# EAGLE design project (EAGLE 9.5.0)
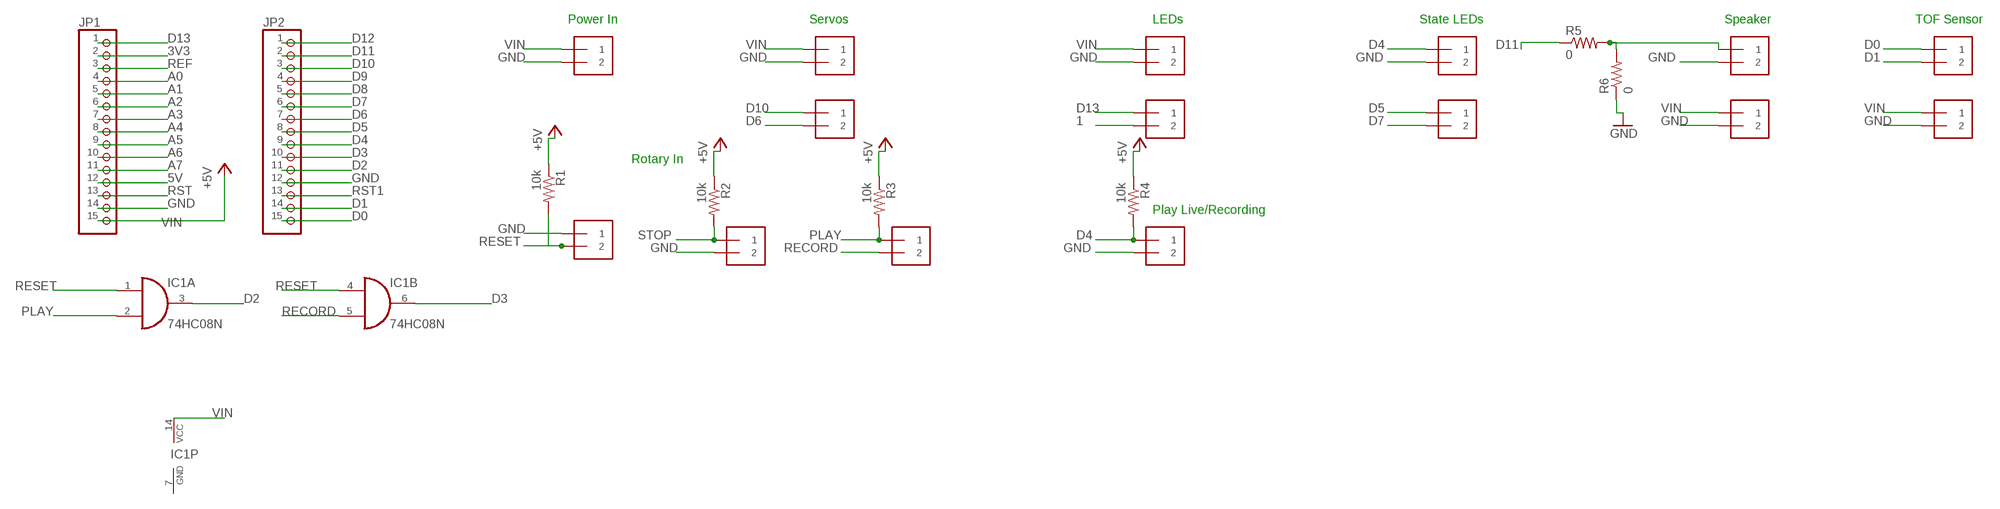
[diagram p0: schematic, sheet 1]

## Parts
IC1  74HC08N  [DIL14]
J1  1X2-3.5MM  [1X2-3.5MM]
J2  1X2-3.5MM  [1X2-3.5MM]
J3  1X2-3.5MM  [1X2-3.5MM]
J4  1X2-3.5MM  [1X2-3.5MM]
JP1  PINHD-1X15  [1X15]
JP2  PINHD-1X15  [1X15]
LED1  1X2-3.5MM  [1X2-3.5MM]
LED2_3  1X2-3.5MM  [1X2-3.5MM]
LED_PWR  1X2-3.5MM  [1X2-3.5MM]
LED_SIG  1X2-3.5MM  [1X2-3.5MM]
POWER  1X2-3.5MM  [1X2-3.5MM]
R1  10k  R-US_M0805  [M0805]
R2  10k  R-US_M0805  [M0805]
R3  10k  R-US_M0805  [M0805]
R4  10k  R-US_M0805  [M0805]
R5  0  R-US_M0805  [M0805]
R6  0  R-US_M0805  [M0805]
SERVO_PWR  1X2-3.5MM  [1X2-3.5MM]
SERVO_SIG  1X2-3.5MM  [1X2-3.5MM]
SPK_PWR  1X2-3.5MM  [1X2-3.5MM]
SPK_SIG  1X2-3.5MM  [1X2-3.5MM]
TOF_PWR  1X2-3.5MM  [1X2-3.5MM]
TOF_SIG  1X2-3.5MM  [1X2-3.5MM]

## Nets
1: LED_SIG.2
3V3: JP1.2
5V: JP1.12
A0: JP1.4
A1: JP1.5
A2: JP1.6
A3: JP1.7
A4: JP1.8
A5: JP1.9
A6: JP1.10
A7: JP1.11
D0: JP2.15 TOF_SIG.1
D1: JP2.14 TOF_SIG.2
D2: IC1.3(A:O) JP2.11
D3: IC1.6(B:O) JP2.10
D4: J1.1 JP2.9 LED1.1 R4.2
D5: JP2.8 LED2_3.1
D6: JP2.7 SERVO_SIG.2
D7: JP2.6 LED2_3.2
D8: JP2.5
D9: JP2.4
D10: JP2.3 SERVO_SIG.1
D11: JP2.2 R5.1
D12: JP2.1
D13: JP1.1 LED_SIG.1
GND: J1.2 J3.2 J4.1 JP1.14 JP2.12 LED1.2 LED_PWR.2 POWER.2 R6.1 SERVO_PWR.2 SPK_PWR.2 SPK_SIG.2 TOF_PWR.2
N$1: R5.2 R6.2 SPK_SIG.1
PLAY: IC1.2(A:I1) J2.1 R3.2
RECORD: IC1.5(B:I1) J2.2
REF: JP1.3
RESET: IC1.1(A:I0) IC1.4(B:I0) J4.2 R1.2
RST: JP1.13
RST1: JP2.13
STOP: J3.1 R2.2
VIN: IC1.14(P:VCC) JP1.15 LED_PWR.1 POWER.1 R1.1 R2.1 R3.1 R4.1 SERVO_PWR.1 SPK_PWR.1 TOF_PWR.1 ; supply symbol labelled +5V
Unconnected: IC1.8(C:O) IC1.9(C:I0) IC1.10(C:I1) IC1.11(D:O) IC1.12(D:I0) IC1.13(D:I1)

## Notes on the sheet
- Power In | Servos | LEDs | State LEDs | Speaker | TOF Sensor
- Rotary In
- Play Live/Recording

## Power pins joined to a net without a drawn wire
GND: IC1.7(P:GND)

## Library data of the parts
IC1 = 74xx-eu:74*08: Quad 2-input AND gate
J1-J4 LED1 LED2_3 LED_PWR LED_SIG POWER SERVO_PWR SERVO_SIG SPK_PWR SPK_SIG TOF_PWR TOF_SIG = adafruit:1X2: 3.5mm Terminal block
JP1 JP2 = adafruit:PINHD-1X15: PIN HEADER
R1-R6 = adafruit:R-US_: RESISTOR, American symbol

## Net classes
0 default: width 0.305 mm, drill 0.508 mm, clearance 0.254 mm

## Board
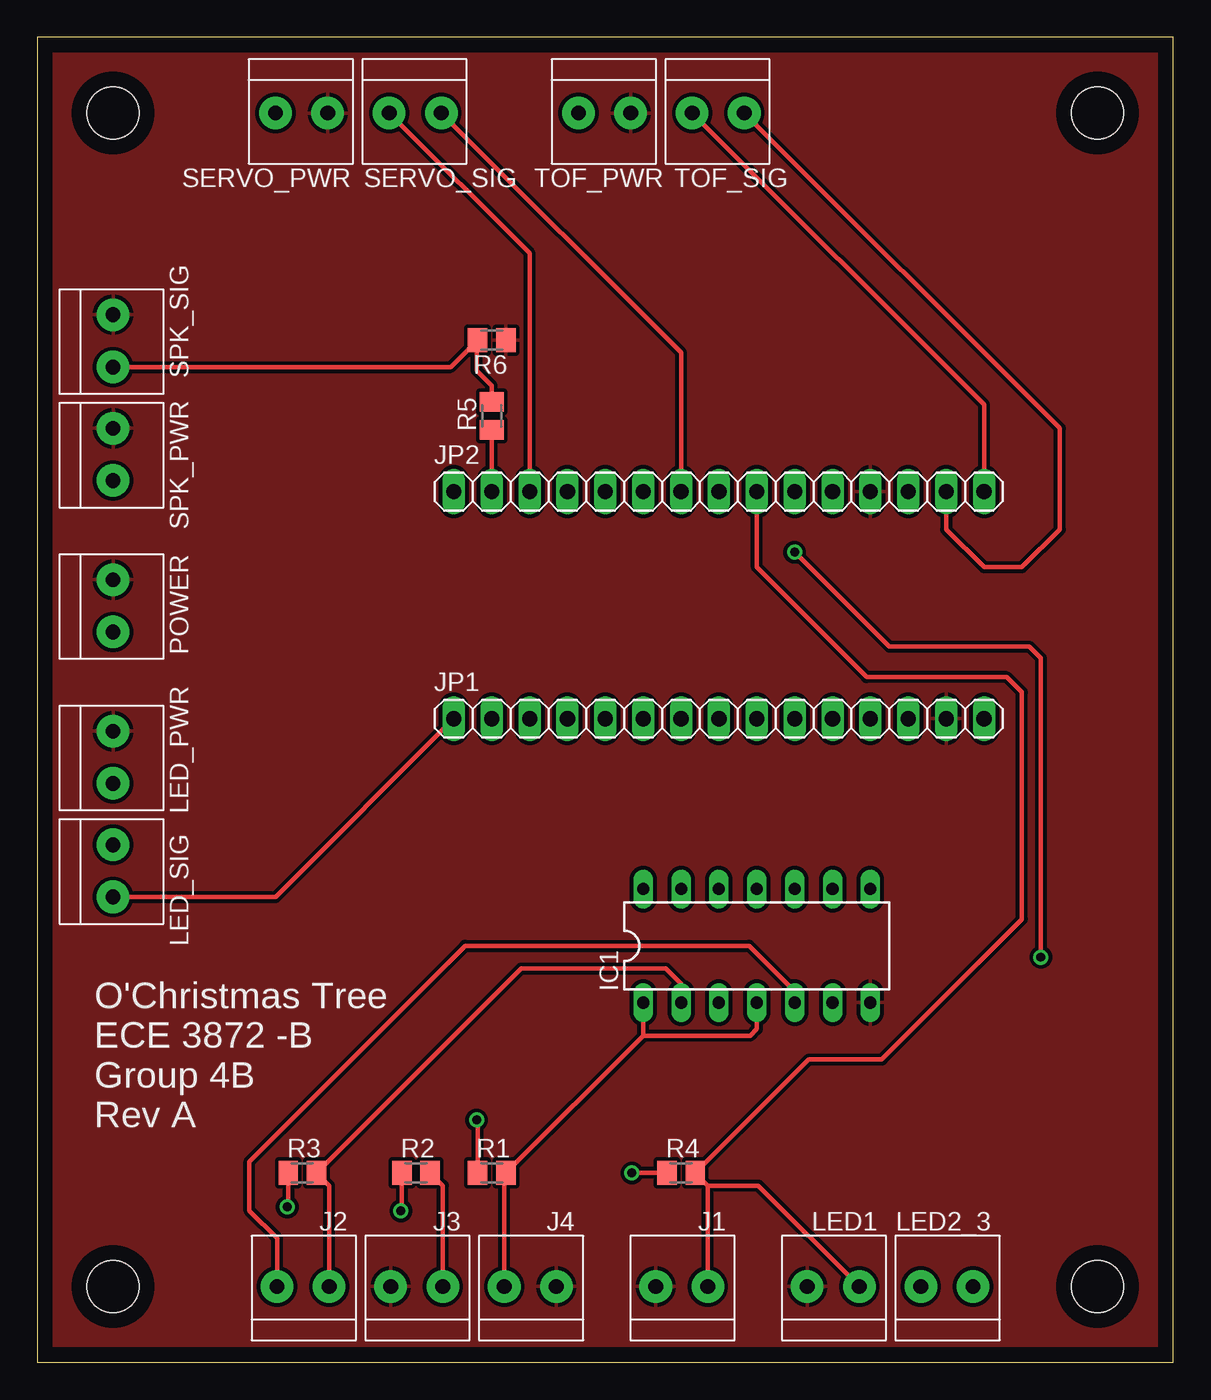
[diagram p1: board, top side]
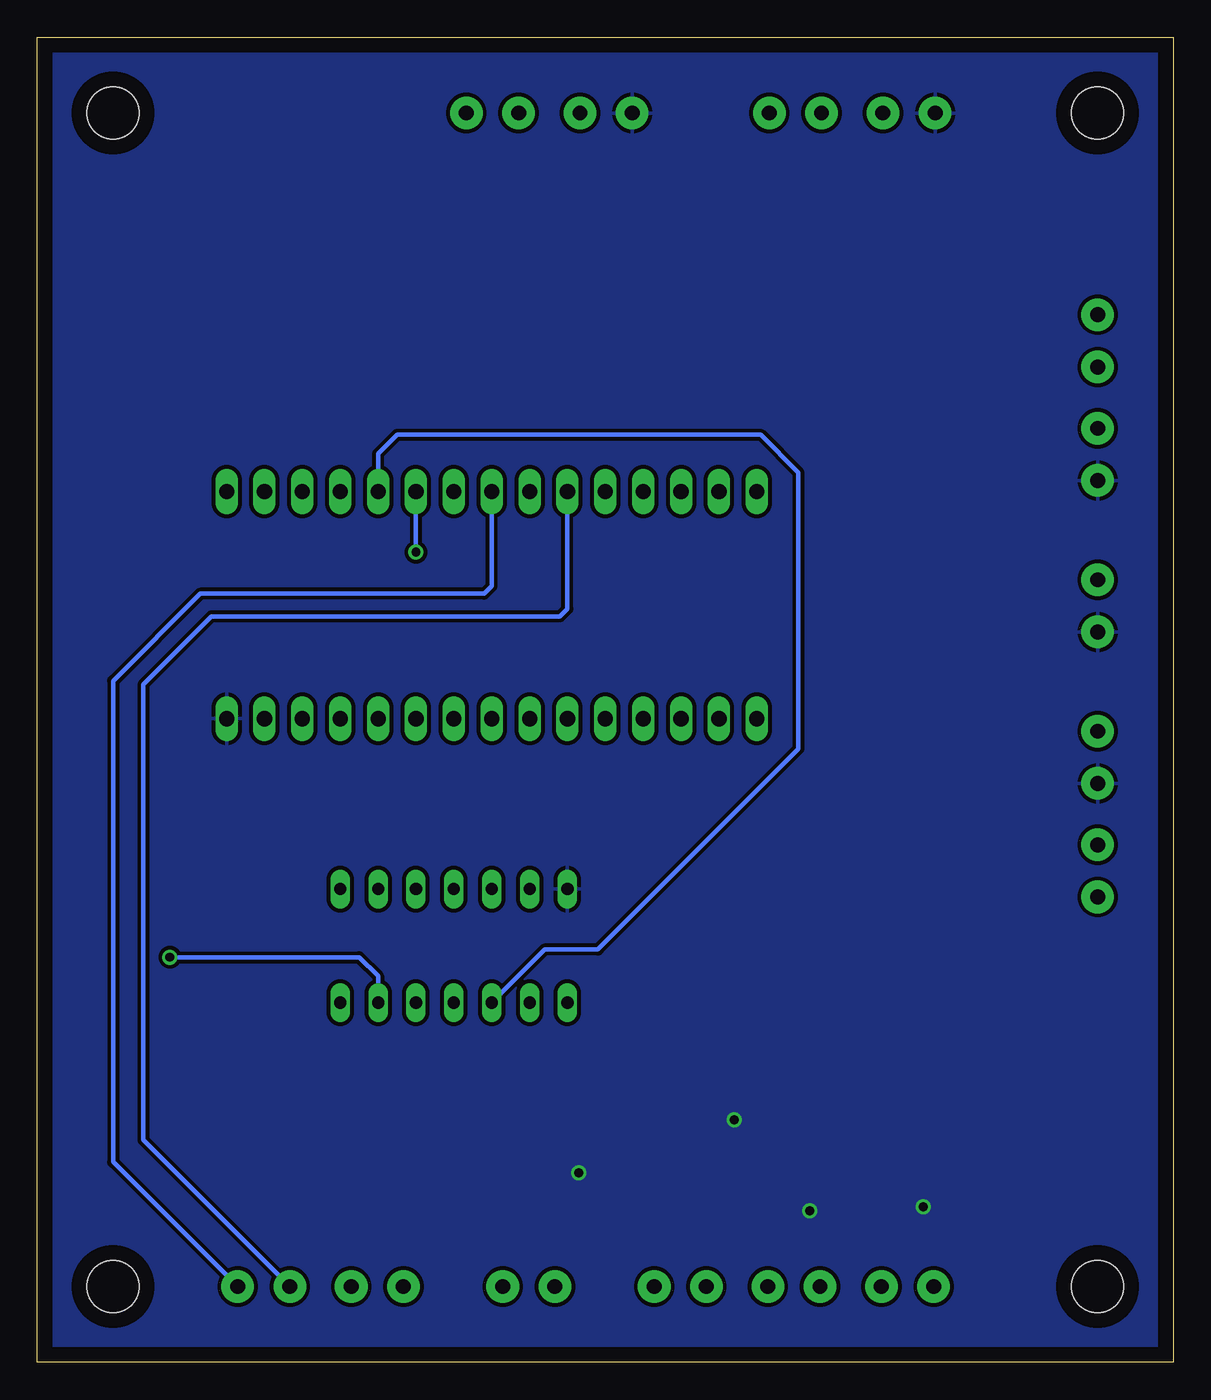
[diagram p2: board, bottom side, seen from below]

Size 76.2 x 88.9 mm. Coordinates in mm from the lower left corner, seen from the top.
Outline: 0,0 76.2,0 76.2,88.9 0,88.9 0,0
Copper layers (1*16): Top 0.035mm / dielectric 1.5mm / Bottom 0.035mm
Design rules "default": minimum track width 6mil, minimum drill 0.35mm, track to track 6mil, track to pad 6mil, pad to pad 6mil, via to via 6mil, smd to smd 6mil, copper to edge 40mil, drill to drill 6mil, minimum pad ring 10mil, minimum via ring 8mil, stop-mask expansion 4mil, vias tented up to drill 0mil, thermal gap 10mil
Holes 3.5 mm at 5.08,5.08 71.12,5.08 71.12,83.82 5.08,83.82

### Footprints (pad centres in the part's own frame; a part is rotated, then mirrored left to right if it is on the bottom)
DIL14 = drill 0.813 long: 1 -7.62,-3.81; 2 -5.08,-3.81; 3 -2.54,-3.81; 4 0,-3.81; 5 2.54,-3.81; 6 5.08,-3.81; 7 7.62,-3.81; 8 7.62,3.81; 9 5.08,3.81; 10 2.54,3.81; 11 0,3.81; 12 -2.54,3.81; 13 -5.08,3.81; 14 -7.62,3.81
1X2-3.5MM = drill 1 pad 2.184: 1 1.8,0; 2 -1.7,0
1X15 = drill 1.016 long: 1 -17.78,0; 2 -15.24,0; 3 -12.7,0; 4 -10.16,0; 5 -7.62,0; 6 -5.08,0; 7 -2.54,0; 8 0,0; 9 2.54,0; 10 5.08,0; 11 7.62,0; 12 10.16,0; 13 12.7,0; 14 15.24,0; 15 17.78,0
M0805 = smd 1.3 x 1.6: 1 -0.95,0; 2 0.95,0

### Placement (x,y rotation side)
IC1  48.26,27.94 0 top
J1  43.18,5.08 0 top
J2  17.78,5.08 0 top
J3  25.4,5.08 0 top
J4  33.02,5.08 0 top
JP1  45.72,43.18 0 top
JP2  45.72,58.42 0 top
LED1  53.34,5.08 0 top
LED2_3  60.96,5.08 0 top
LED_PWR  5.08,40.64 270 top
LED_SIG  5.08,33.02 270 top
POWER  5.08,50.8 270 top
R1  30.48,12.7 0 top
R2  25.4,12.7 0 top
R3  17.78,12.7 0 top
R4  43.18,12.7 0 top
R5  30.48,63.5 90 top
R6  30.48,68.58 180 top
SERVO_PWR  17.78,83.82 180 top
SERVO_SIG  25.4,83.82 180 top
SPK_PWR  5.08,60.96 270 top
SPK_SIG  5.08,68.58 270 top
TOF_PWR  38.1,83.82 180 top
TOF_SIG  45.72,83.82 180 top

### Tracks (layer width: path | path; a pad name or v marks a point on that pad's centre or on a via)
D0
  Top 0.305: JP2.15 63.5,64.24 TOF_SIG.1
D1
  Top 0.305: JP2.14 60.96,55.88 63.5,53.34 66.04,53.34 68.58,55.88 68.58,62.66 TOF_SIG.2
D2
  Bottom 0.305: JP2.11 53.34,60.96 52.07,62.23 27.69,62.23 25.15,59.69 25.15,41.15 38.61,27.69 42.16,27.69 IC1.3
D3  (via drill 0.6)
  Top 0.305: v50.8,54.36 57.15,48.01 66.55,48.01 67.31,47.24 v67.31,27.18
  Bottom 0.305: JP2.10 v50.8,54.36 | v67.31,27.18 54.61,27.18 53.34,25.91 IC1.6
D4
  Top 0.305: J1.1 44.98,11.85 | 44.98,11.85 R4.2 51.75,20.32 56.64,20.32 66.04,29.72 66.04,44.96 65.02,45.97 55.63,45.97 48.26,53.34 JP2.9 | LED1.1 48.37,11.85 44.98,11.85
D5
  Bottom 0.305: LED2_3.1 71.12,13.44 71.12,45.72 65.28,51.56 46.23,51.56 45.72,52.07 JP2.8
D6
  Top 0.305: JP2.7 43.18,67.74 SERVO_SIG.2
D7
  Bottom 0.305: LED2_3.2 69.09,14.91 69.09,45.47 64.52,50.04 41.15,50.04 40.64,50.55 JP2.6
D10
  Top 0.305: SERVO_SIG.1 33.02,74.4 JP2.3
D11
  Top 0.305: JP2.2 R5.1
D13
  Top 0.305: LED_SIG.1 15.98,31.22 JP1.1
GND
  pour Top: -2.54,91.44 -2.54,-2.54 78.74,-2.54 78.74,91.44
N$1
  Top 0.305: SPK_SIG.1 27.73,66.78 R6.2 29.46,68.51 29.46,66.55 30.48,65.53 R5.2
PLAY
  Top 0.305: J2.1 19.58,11.85 R3.2 32.45,26.42 42.16,26.42 43.18,25.4 IC1.2
RECORD
  Top 0.305: J2.2 16.08,8.3 14.22,10.16 14.22,13.46 28.7,27.94 47.75,27.94 50.8,24.89 IC1.5
RESET
  Top 0.305: J4.2 31.32,12.59 R1.2 40.64,21.91 | 40.64,21.91 IC1.1 | IC1.4 48.26,22.35 47.82,21.91 40.64,21.91
STOP
  Top 0.305: J3.1 27.2,11.85 R2.2
VIN  (via drill 0.6)
  Top 0.305: R3.1 16.83,10.48 v16.76,10.41 | R2.1 24.45,10.23 v24.38,10.16 | R1.1 29.53,16.19 v29.46,16.26 | R4.1 v39.88,12.7
  pour Bottom: -2.54,91.44 -2.54,-2.54 78.74,-2.54 78.74,91.44

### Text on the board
_tsilk: O'Christmas Tree / ECE 3872 -B / Group 4B / Rev A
